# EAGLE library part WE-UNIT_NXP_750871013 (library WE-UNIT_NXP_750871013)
Off-Line Transformer WE-Unit NXP - Nominal input voltage: 85-265 VAC - Operating temperature: -40°C to +125 °C - Isolation voltage 4 kVAC -- Especially designed for several ICs from NXP TEA1521T -- Universal input -- Smart meters -- Dimmable 12 V LED driver -- Offline-switch mode power supplies
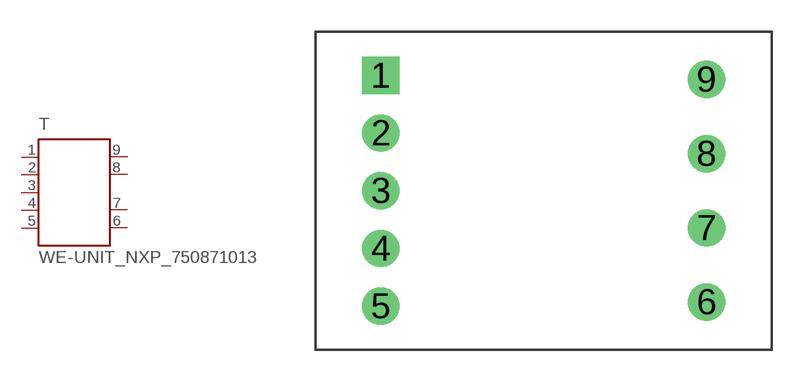
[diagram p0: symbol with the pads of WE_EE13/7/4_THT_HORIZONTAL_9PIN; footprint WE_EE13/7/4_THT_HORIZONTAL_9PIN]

Designator prefix T

## WE-UNIT_NXP_750871013 (MPN: 750871013; OC_FARNELL: 1849052; OC_NEWARK: 13T9840; PACKAGE: EE13_7_4_NXP; SUPPLIER: Würth Elektronik eiSos GmbH)  [WE_EE13/7/4_THT_HORIZONTAL_9PIN]
1  5  pas
2  4  pas
3  3  pas
4  2  pas
5  1  pas
6  9  pas
7  8  pas
8  7  pas
9  6  pas

## Footprint WE_EE13/7/4_THT_HORIZONTAL_9PIN (pad centres in mm)
Transformer, EE13/7/4 THT Horizontal 9 Pins
drill 1.17 square: 1 -7.675,5.44
drill 1.17: 2 -7.675,2.72; 3 -7.675,0; 4 -7.675,-2.72; 5 -7.675,-5.44; 6 7.675,-5.25; 7 7.675,-1.75; 8 7.675,1.75; 9 7.675,5.25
